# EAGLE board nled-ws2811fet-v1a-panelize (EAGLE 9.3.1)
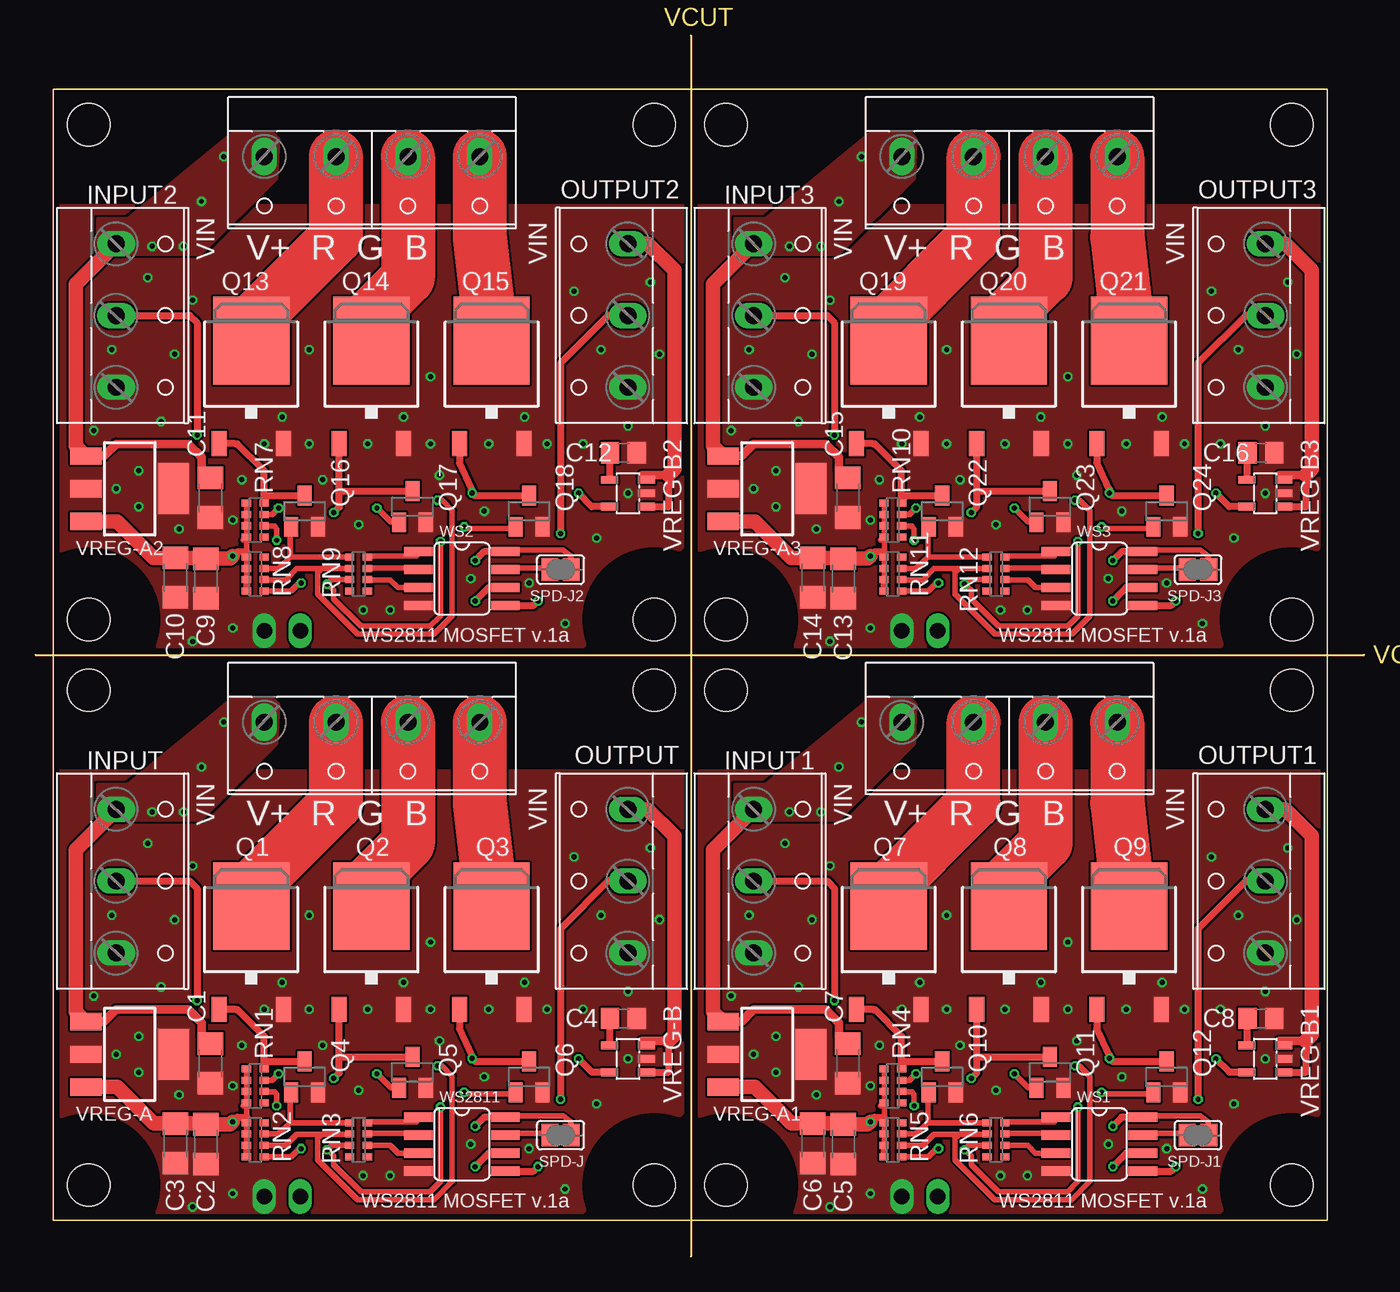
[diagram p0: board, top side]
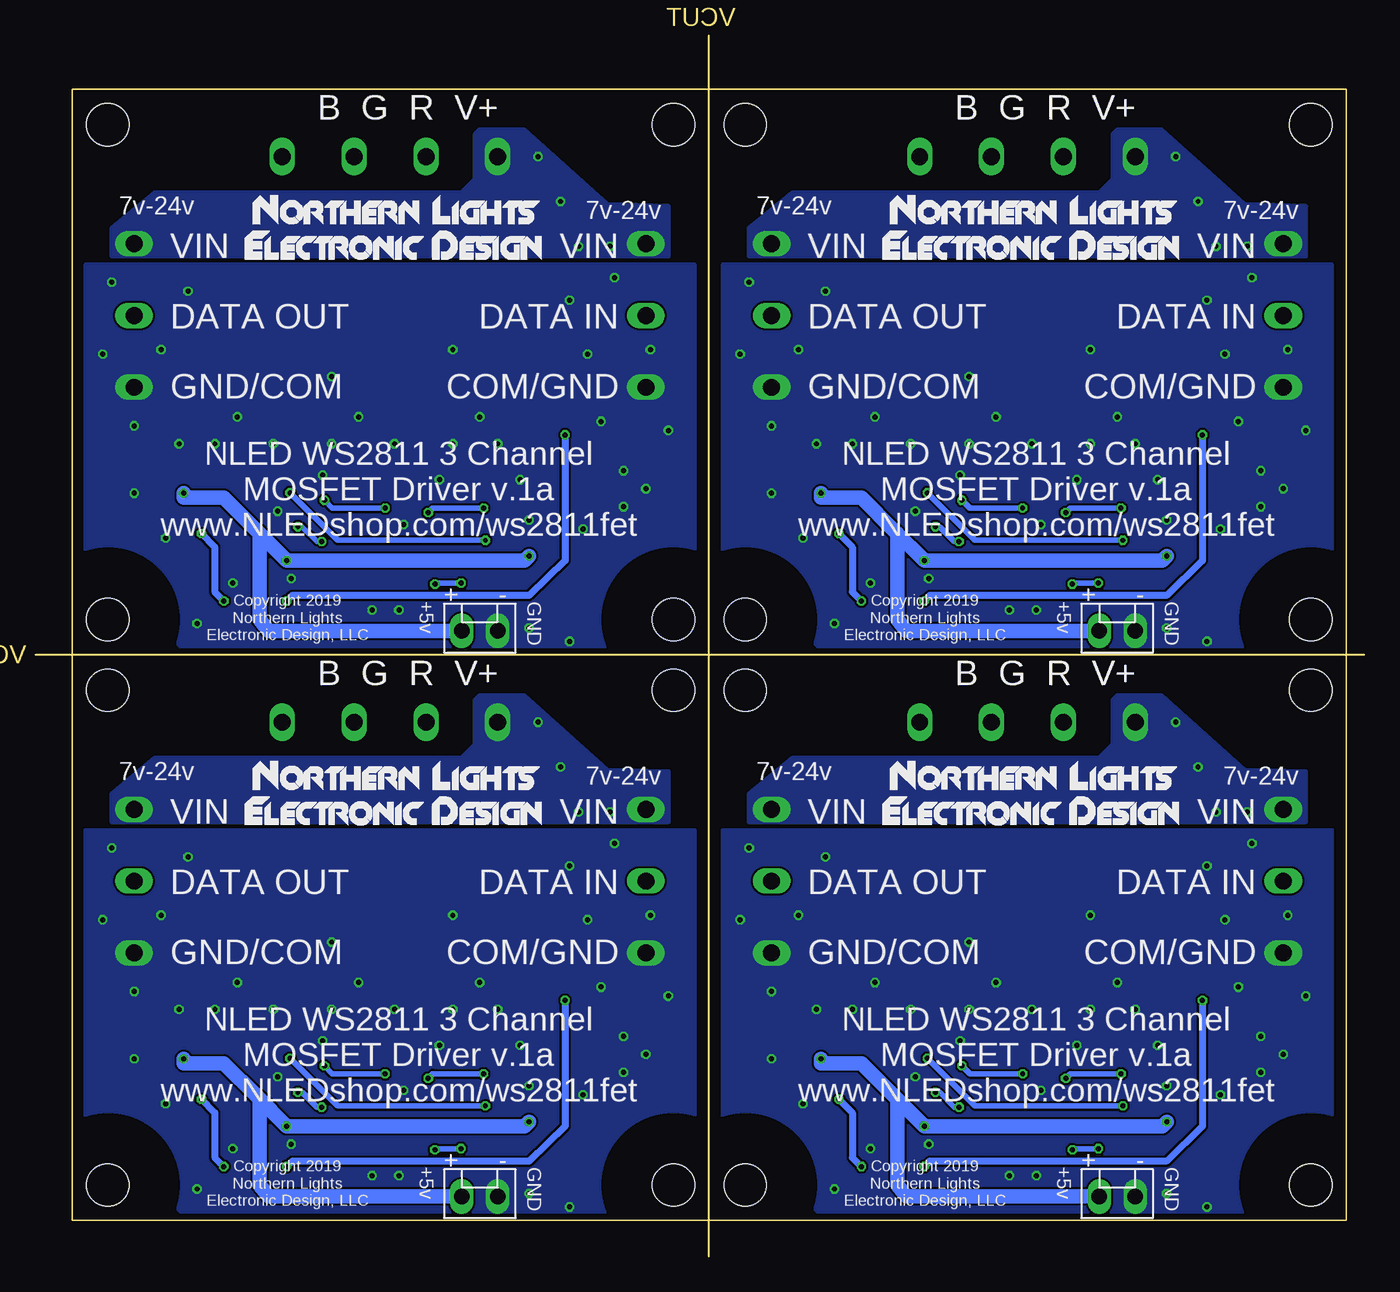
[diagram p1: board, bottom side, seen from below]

Size 93.98 x 86.36 mm. Coordinates in mm from the lower left corner, seen from the top.
Outline: 46.27,2.54 1.27,2.54 1.27,82.55
Outline: 46.36,2.54 91.35,2.54 91.35,82.55 1.27,82.55
Outline: 46.36,86.36 46.36,0
Outline: 0,42.54 93.98,42.54
Copper layers (1*2*15*16): Top 0.035mm / dielectric 0.2mm / Route2 0.0175mm / dielectric 1.1mm / Route15 0.0175mm / dielectric 0.2mm / Bottom 0.035mm
Design rules "SeeedStudio_DRU_no_angle_20130527 *": minimum track width 6mil, minimum drill 12mil, track to track 6mil, track to pad 12mil, pad to pad 6mil, via to via 6mil, smd to smd 0mil, copper to edge 16mil, drill to drill 10mil, minimum pad ring 6mil, minimum via ring 6mil, stop-mask expansion 2mil, vias tented up to drill 25mil, thermal gap 10mil
Net classes: 0 default: width 0.406 mm
Holes 3 mm at 3.77,5.04 43.77,40.04 3.77,40.04 43.77,5.04 48.86,5.04 88.85,40.04 48.86,40.04 88.85,5.04 3.77,45.05 43.77,80.05 3.77,80.05 43.77,45.05 48.86,45.05 88.85,80.05 48.86,80.05 88.85,45.05
tRestrict: area -1.2,35 to 8.8,45; area -1.2,0 to 8.8,10; area 38.8,35 to 48.8,45; area 38.8,0 to 48.8,10; area 43.9,35 to 53.9,45; area 43.9,0 to 53.9,10; area 83.9,35 to 93.9,45; area 83.9,0 to 93.9,10; area -1.2,75 to 8.8,85; area -1.2,40 to 8.8,50; area 38.8,75 to 48.8,85; area 38.8,40 to 48.8,50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
bRestrict: area -1.2,0 to 8.8,10; area -1.2,35 to 8.8,45; area 38.8,35 to 48.8,45; area 38.8,0 to 48.8,10; area 43.9,0 to 53.9,10; area 43.9,35 to 53.9,45; area 83.9,35 to 93.9,45; area 83.9,0 to 93.9,10; area -1.2,40 to 8.8,50; area -1.2,75 to 8.8,85; area 38.8,75 to 48.8,85; area 38.8,40 to 48.8,50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

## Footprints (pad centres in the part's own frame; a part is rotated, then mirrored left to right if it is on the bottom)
MOLEXKK2PWR = drill 1.1 long: 1 -1.27,0; 2 1.27,0
C1206 = smd 1.6 x 1.8: 1 -1.4,0; 2 1.4,0
C0805 = smd 1.3 x 1.5: 1 -0.95,0; 2 0.95,0
W237-133 = drill 1.194 long: 1 -5.08,-0.635; 2 0,-0.635; 3 5.08,-0.635
W237-4P = drill 1.194 long: 1 -7.62,-0.635; 2 -2.54,-0.635; 3 2.54,-0.635; 4 7.62,-0.635
DPAK-2PIN = smd 1.067 x 1.778: 1 -2.28,-6.07; 3 2.28,-6.07 | smd 5.4 x 6.2: 2 0,1.23
SOT23 = smd 1 x 1.4: 1 -0.95,-1.1; 2 0.95,-1.1; 3 0,1.1
0603-ARV = smd 0.5 x 0.65: 1 -1.2,-0.625; 2 -0.4,-0.625; 3 0.4,-0.625; 4 1.2,-0.625; 5 1.2,0.625; 6 0.4,0.625; 7 -0.4,0.625; 8 -1.2,0.625
SJ = smd 1.168 x 1.6: 1 -0.762,0; 2 0.762,0
SOT223 = smd 1.219 x 2.235: 1 -2.311,-3.099; 2 0,-3.099; 3 2.311,-3.099 | smd 3.6 x 2.2: 4 0,3.099
SOT25 = smd 0.55 x 1.2: 1 -0.95,-1.3; 2 0,-1.3; 3 0.95,-1.3; 4 0.95,1.3; 5 -0.95,1.3
SOIC-8 = smd 0.66 x 2.032: 1 -1.905,-3.073; 2 -0.635,-3.073; 3 0.635,-3.073; 4 1.905,-3.073; 5 1.905,3.073; 6 0.635,3.073; 7 -0.635,3.073; 8 -1.905,3.073

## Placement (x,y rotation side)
5VOUT  MOLEX-KK-2P5V  [MOLEXKK2PWR]  17.46,4.24 0 bottom
5VOUT1  MOLEX-KK-2P5V  [MOLEXKK2PWR]  62.55,4.24 0 bottom
5VOUT2  MOLEX-KK-2P5V  [MOLEXKK2PWR]  17.46,44.24 0 bottom
5VOUT3  MOLEX-KK-2P5V  [MOLEXKK2PWR]  62.55,44.24 0 bottom
C1  0.1uF, >24v  [C1206]  12.38,13.65 270 top
C2  0.1uF, >6.3vdc  [C1206]  12.06,7.94 270 top
C3  10uF, >6.3vdc  [C1206]  9.91,8 270 top
C4  100pF  [C0805]  41.59,16.83 0 top
C5  0.1uF, >6.3vdc  [C1206]  57.15,7.94 270 top
C6  10uF, >6.3vdc  [C1206]  54.99,8 270 top
C7  0.1uF, >24v  [C1206]  57.47,13.65 270 top
C8  100pF  [C0805]  86.68,16.83 0 top
C9  0.1uF, >6.3vdc  [C1206]  12.06,47.94 270 top
C10  10uF, >6.3vdc  [C1206]  9.91,48.01 270 top
C11  0.1uF, >24v  [C1206]  12.38,53.66 270 top
C12  100pF  [C0805]  41.59,56.83 0 top
C13  0.1uF, >6.3vdc  [C1206]  57.15,47.94 270 top
C14  10uF, >6.3vdc  [C1206]  54.99,48.01 270 top
C15  0.1uF, >24v  [C1206]  57.47,53.66 270 top
C16  100pF  [C0805]  86.68,56.83 0 top
INPUT  [W237-133]  6.35,26.54 270 top
INPUT1  [W237-133]  51.44,26.54 270 top
INPUT2  [W237-133]  6.35,66.55 270 top
INPUT3  [W237-133]  51.44,66.55 270 top
LEDOUT  [W237-4P]  23.81,37.15 180 top
LEDOUT1  [W237-4P]  68.9,37.15 180 top
LEDOUT2  [W237-4P]  23.81,77.15 180 top
LEDOUT3  [W237-4P]  68.9,77.15 180 top
OUTPUT  [W237-133]  41.28,26.54 90 top
OUTPUT1  [W237-133]  86.36,26.54 90 top
OUTPUT2  [W237-133]  41.28,66.55 90 top
OUTPUT3  [W237-133]  86.36,66.55 90 top
Q1  NCHAN-DPAK-2  [DPAK-2PIN]  15.27,23.54 0 top
Q2  NCHAN-DPAK-2  [DPAK-2PIN]  23.77,23.54 0 top
Q3  NCHAN-DPAK-2  [DPAK-2PIN]  32.27,23.54 0 top
Q4  BSS123  [SOT23]  19.05,12.7 0 top
Q5  BSS123  [SOT23]  26.67,13.02 0 top
Q6  BSS123  [SOT23]  34.93,12.7 0 top
Q7  NCHAN-DPAK-2  [DPAK-2PIN]  60.36,23.54 0 top
Q8  NCHAN-DPAK-2  [DPAK-2PIN]  68.85,23.54 0 top
Q9  NCHAN-DPAK-2  [DPAK-2PIN]  77.35,23.54 0 top
Q10  BSS123  [SOT23]  64.14,12.7 0 top
Q11  BSS123  [SOT23]  71.75,13.02 0 top
Q12  BSS123  [SOT23]  80.01,12.7 0 top
Q13  NCHAN-DPAK-2  [DPAK-2PIN]  15.27,63.55 0 top
Q14  NCHAN-DPAK-2  [DPAK-2PIN]  23.77,63.55 0 top
Q15  NCHAN-DPAK-2  [DPAK-2PIN]  32.27,63.55 0 top
Q16  BSS123  [SOT23]  19.05,52.7 0 top
Q17  BSS123  [SOT23]  26.67,53.02 0 top
Q18  BSS123  [SOT23]  34.93,52.7 0 top
Q19  NCHAN-DPAK-2  [DPAK-2PIN]  60.36,63.55 0 top
Q20  NCHAN-DPAK-2  [DPAK-2PIN]  68.85,63.55 0 top
Q21  NCHAN-DPAK-2  [DPAK-2PIN]  77.35,63.55 0 top
Q22  BSS123  [SOT23]  64.14,52.7 0 top
Q23  BSS123  [SOT23]  71.75,53.02 0 top
Q24  BSS123  [SOT23]  80.01,52.7 0 top
RN1  10k  [0603-ARV]  15.56,12.07 90 top
RN2  10k  [0603-ARV]  15.56,8.25 90 top
RN3  100  [0603-ARV]  22.86,8.25 270 top
RN4  10k  [0603-ARV]  60.64,12.07 90 top
RN5  10k  [0603-ARV]  60.64,8.25 90 top
RN6  100  [0603-ARV]  67.94,8.25 270 top
RN7  10k  [0603-ARV]  15.56,52.07 90 top
RN8  10k  [0603-ARV]  15.56,48.26 90 top
RN9  100  [0603-ARV]  22.86,48.26 270 top
RN10  10k  [0603-ARV]  60.64,52.07 90 top
RN11  10k  [0603-ARV]  60.64,48.26 90 top
RN12  100  [0603-ARV]  67.94,48.26 270 top
SPD-J  [SJ]  37.15,8.57 0 top
SPD-J1  [SJ]  82.23,8.57 0 top
SPD-J2  [SJ]  37.15,48.58 0 top
SPD-J3  [SJ]  82.23,48.58 0 top
VREG-A  UA78M05DCY  [SOT223]  6.67,14.29 270 top
VREG-A1  UA78M05DCY  [SOT223]  51.75,14.29 270 top
VREG-A2  UA78M05DCY  [SOT223]  6.67,54.29 270 top
VREG-A3  UA78M05DCY  [SOT223]  51.75,54.29 270 top
VREG-B  AP2210K  [SOT25]  41.91,13.97 90 top
VREG-B1  AP2210K  [SOT25]  86.99,13.97 90 top
VREG-B2  AP2210K  [SOT25]  41.91,53.98 90 top
VREG-B3  AP2210K  [SOT25]  86.99,53.98 90 top
WS1  WS2811  [SOIC-8]  75.25,7.94 270 top
WS2  WS2811  [SOIC-8]  30.16,47.94 270 top
WS3  WS2811  [SOIC-8]  75.25,47.94 270 top
WS2811  WS2811  [SOIC-8]  30.16,7.94 270 top

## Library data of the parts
5VOUT 5VOUT1-5VOUT3 = NLED-connectors
C1-C3 C5-C7 C9-C11 C13-C15 = rcl
C4 C8 C12 C16 = rcl; SPICEPREFIX: C
INPUT INPUT1-INPUT3 LEDOUT LEDOUT1-LEDOUT3 OUTPUT OUTPUT1-OUTPUT3 = con-wago-508; OC_FARNELL: unknown; OC_NEWARK: unknown
Q1-Q3 Q7-Q9 Q13-Q15 Q19-Q21 VREG-A VREG-A1-VREG-A3 VREG-B VREG-B1-VREG-B3 WS1-WS3 WS2811 = NLED-integratedcircuit
Q4-Q6 Q10-Q12 Q16-Q18 Q22-Q24 = transistor-small-signal
RN1-RN12 = resistor-dil; OC_FARNELL: unknown; OC_NEWARK: unknown
SPD-J SPD-J1-SPD-J3 = NLED-misc

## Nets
BINV: Q3.1 Q6.3 RN1.2
BINV1: Q9.1 Q12.3 RN4.2
BINV2: Q15.1 Q18.3 RN7.2
BINV3: Q21.1 Q24.3 RN10.2
BYPASS: C4.1 VREG-B.4
BYPASS1: C8.1 VREG-B1.4
BYPASS2: C12.1 VREG-B2.4
BYPASS3: C16.1 VREG-B3.4
DIN: INPUT.2 WS2811.6
DIN1: INPUT1.2 WS1.6
DIN2: INPUT2.2 WS2.6
DIN3: INPUT3.2 WS3.6
DOUT: OUTPUT.2 WS2811.5
DOUT1: OUTPUT1.2 WS1.5
DOUT2: OUTPUT2.2 WS2.5
DOUT3: OUTPUT3.2 WS3.5
GINV: Q2.1 Q5.3 RN1.3
GINV1: Q8.1 Q11.3 RN4.3
GINV2: Q14.1 Q17.3 RN7.3
GINV3: Q20.1 Q23.3 RN10.3
GND: 5VOUT.2 C1.2 C2.2 C3.2 C4.2 INPUT.3 OUTPUT.1 Q1.3 Q2.3 Q3.3 Q4.2 Q5.2 Q6.2 VREG-A.2 VREG-A.4 VREG-B.2 WS2811.4
GND1: 5VOUT1.2 C5.2 C6.2 C7.2 C8.2 INPUT1.3 OUTPUT1.1 Q7.3 Q8.3 Q9.3 Q10.2 Q11.2 Q12.2 VREG-A1.2 VREG-A1.4 VREG-B1.2 WS1.4
GND2: 5VOUT2.2 C9.2 C10.2 C11.2 C12.2 INPUT2.3 OUTPUT2.1 Q13.3 Q14.3 Q15.3 Q16.2 Q17.2 Q18.2 VREG-A2.2 VREG-A2.4 VREG-B2.2 WS2.4
GND3: 5VOUT3.2 C13.2 C14.2 C15.2 C16.2 INPUT3.3 OUTPUT3.1 Q19.3 Q20.3 Q21.3 Q22.2 Q23.2 Q24.2 VREG-A3.2 VREG-A3.4 VREG-B3.2 WS3.4
N$1: SPD-J1.1 WS1.7
N$2: RN6.8 WS1.1
N$3: RN3.8 WS2811.1
N$4: RN6.7 WS1.2
N$5: RN3.7 WS2811.2
N$6: RN6.6 WS1.3
N$7: RN3.6 WS2811.3
N$8: SPD-J2.1 WS2.7
N$9: RN9.8 WS2.1
N$10: RN9.7 WS2.2
N$11: RN9.6 WS2.3
N$12: SPD-J3.1 WS3.7
N$13: SPD-J.1 WS2811.7
N$14: RN12.8 WS3.1
N$15: RN12.7 WS3.2
N$16: RN12.6 WS3.3
OUTB-1: Q6.1 RN2.1 RN3.3
OUTB-2: Q12.1 RN5.1 RN6.3
OUTB-3: Q18.1 RN8.1 RN9.3
OUTB-4: Q24.1 RN11.1 RN12.3
OUTBLUE: LEDOUT.3 Q1.2
OUTBLUE1: LEDOUT1.3 Q7.2
OUTBLUE2: LEDOUT2.3 Q13.2
OUTBLUE3: LEDOUT3.3 Q19.2
OUTG-1: Q5.1 RN2.2 RN3.2
OUTG-2: Q11.1 RN5.2 RN6.2
OUTG-3: Q17.1 RN8.2 RN9.2
OUTG-4: Q23.1 RN11.2 RN12.2
OUTGREEN: LEDOUT.2 Q2.2
OUTGREEN1: LEDOUT1.2 Q8.2
OUTGREEN2: LEDOUT2.2 Q14.2
OUTGREEN3: LEDOUT3.2 Q20.2
OUTR-1: Q4.1 RN2.3 RN3.1
OUTR-2: Q10.1 RN5.3 RN6.1
OUTR-3: Q16.1 RN8.3 RN9.1
OUTR-4: Q22.1 RN11.3 RN12.1
OUTRED: LEDOUT.1 Q3.2
OUTRED1: LEDOUT1.1 Q9.2
OUTRED2: LEDOUT2.1 Q15.2
OUTRED3: LEDOUT3.1 Q21.2
RINV: Q1.1 Q4.3 RN1.4
RINV1: Q7.1 Q10.3 RN4.4
RINV2: Q13.1 Q16.3 RN7.4
RINV3: Q19.1 Q22.3 RN10.4
VCC: 5VOUT.1 C2.1 C3.1 RN1.5 RN1.6 RN1.7 RN1.8 RN2.5 RN2.6 RN2.7 RN2.8 SPD-J.2 VREG-A.3 VREG-B.5 WS2811.8
VCC1: 5VOUT1.1 C5.1 C6.1 RN4.5 RN4.6 RN4.7 RN4.8 RN5.5 RN5.6 RN5.7 RN5.8 SPD-J1.2 VREG-A1.3 VREG-B1.5 WS1.8
VCC2: 5VOUT2.1 C9.1 C10.1 RN7.5 RN7.6 RN7.7 RN7.8 RN8.5 RN8.6 RN8.7 RN8.8 SPD-J2.2 VREG-A2.3 VREG-B2.5 WS2.8
VCC3: 5VOUT3.1 C13.1 C14.1 RN10.5 RN10.6 RN10.7 RN10.8 RN11.5 RN11.6 RN11.7 RN11.8 SPD-J3.2 VREG-A3.3 VREG-B3.5 WS3.8
VIN: C1.1 INPUT.1 LEDOUT.4 OUTPUT.3 VREG-A.1 VREG-B.1 VREG-B.3
VIN1: C7.1 INPUT1.1 LEDOUT1.4 OUTPUT1.3 VREG-A1.1 VREG-B1.1 VREG-B1.3
VIN2: C11.1 INPUT2.1 LEDOUT2.4 OUTPUT2.3 VREG-A2.1 VREG-B2.1 VREG-B2.3
VIN3: C15.1 INPUT3.1 LEDOUT3.4 OUTPUT3.3 VREG-A3.1 VREG-B3.1 VREG-B3.3

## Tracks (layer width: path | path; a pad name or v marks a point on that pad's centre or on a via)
BINV  (via drill 0.35)
  Top 0.406: RN1.2 16.32,11.64 16.92,11.64 17.07,11.45 v17.07,10.64
  Top 0.508: Q3.1 29.99,16.13 30.89,14.23 v30.89,14 31.08,13.8 Q6.3
  Bottom 0.406: v17.07,10.64 27.53,10.64 v30.89,14
BINV1  (via drill 0.35)
  Top 0.406: RN4.2 61.4,11.64 62,11.64 62.16,11.45 v62.16,10.64
  Top 0.508: Q9.1 75.08,16.13 75.97,14.23 v75.97,14 76.17,13.8 Q12.3
  Bottom 0.406: v62.16,10.64 72.62,10.64 v75.97,14
BINV2  (via drill 0.35)
  Top 0.406: RN7.2 16.32,51.64 16.92,51.64 17.07,51.45 v17.07,50.65
  Top 0.508: Q15.1 29.99,56.13 30.89,54.23 v30.89,54 31.08,53.8 Q18.3
  Bottom 0.406: v17.07,50.65 27.53,50.65 v30.89,54
BINV3  (via drill 0.35)
  Top 0.406: RN10.2 61.4,51.64 62,51.64 62.16,51.45 v62.16,50.65
  Top 0.508: Q21.1 75.08,56.13 75.97,54.23 v75.97,54 76.17,53.8 Q24.3
  Bottom 0.406: v62.16,50.65 72.62,50.65 v75.97,54
BYPASS
  Top 0.508: VREG-B.4 40.64,14.95 C4.1
BYPASS1
  Top 0.508: VREG-B1.4 85.73,14.95 C8.1
BYPASS2
  Top 0.508: VREG-B2.4 40.64,54.96 C12.1
BYPASS3
  Top 0.508: VREG-B3.4 85.73,54.96 C16.1
DIN  (via drill 0.35)
  Top 0.508: WS2811.6 32.07,7.3 v31.11,6.35 | v11.43,18.1 11.43,26.04 10.92,26.54 INPUT.2
  Bottom 0.508: v11.43,18.1 11.43,9.21 13.97,6.74 26.35,6.74 30.72,6.74 v31.11,6.35
DIN1  (via drill 0.35)
  Top 0.508: WS1.6 77.15,7.3 v76.2,6.35 | v56.52,18.1 56.52,26.04 56.01,26.54 INPUT1.2
  Bottom 0.508: v56.52,18.1 56.52,9.21 59.05,6.74 71.44,6.74 75.81,6.74 v76.2,6.35
DIN2  (via drill 0.35)
  Top 0.508: WS2.6 32.07,47.31 v31.11,46.35 | v11.43,58.1 11.43,66.04 10.92,66.55 INPUT2.2
  Bottom 0.508: v11.43,58.1 11.43,49.21 13.97,46.74 26.35,46.74 30.72,46.74 v31.11,46.35
DIN3  (via drill 0.35)
  Top 0.508: WS3.6 77.15,47.31 v76.2,46.35 | v56.52,58.1 56.52,66.04 56.01,66.55 INPUT3.2
  Bottom 0.508: v56.52,58.1 56.52,49.21 59.05,46.74 71.44,46.74 75.81,46.74 v76.2,46.35
DOUT  (via drill 0.35)
  Top 0.508: WS2811.5 35.24,6.03 v35.56,6.35 | OUTPUT.2 40.51,26.54 37.15,23.18 v37.15,11.11
  Bottom 0.508: v35.56,6.35 36.2,6.99 36.2,10.16 v37.15,11.11
DOUT1  (via drill 0.35)
  Top 0.508: WS1.5 80.33,6.03 v80.64,6.35 | OUTPUT1.2 85.59,26.54 82.23,23.18 v82.23,11.11
  Bottom 0.508: v80.64,6.35 81.28,6.99 81.28,10.16 v82.23,11.11
DOUT2  (via drill 0.35)
  Top 0.508: WS2.5 35.24,46.04 v35.56,46.35 | OUTPUT2.2 40.51,66.55 37.15,63.18 v37.15,51.12
  Bottom 0.508: v35.56,46.35 36.2,46.99 36.2,50.16 v37.15,51.12
DOUT3  (via drill 0.35)
  Top 0.508: WS3.5 80.33,46.04 v80.64,46.35 | OUTPUT3.2 85.59,66.55 82.23,63.18 v82.23,51.12
  Bottom 0.508: v80.64,46.35 81.28,46.99 81.28,50.16 v82.23,51.12
GINV  (via drill 0.35)
  Top 0.406: v17.2,12.92 16.75,12.46 RN1.3
  Top 0.508: v21.11,12.6 21.49,12.98 21.49,13.97 | 21.49,13.97 Q2.1 | 21.49,13.97 21.64,14.12 Q5.3
  Bottom 0.406: v21.11,12.6 20.79,12.92 v17.2,12.92
GINV1  (via drill 0.35)
  Top 0.406: v62.28,12.92 61.83,12.46 RN4.3
  Top 0.508: v66.19,12.6 66.58,12.98 66.58,13.97 | 66.58,13.97 Q8.1 | 66.58,13.97 66.72,14.12 Q11.3
  Bottom 0.406: v66.19,12.6 65.88,12.92 v62.28,12.92
GINV2  (via drill 0.35)
  Top 0.406: v17.2,52.92 16.75,52.47 RN7.3
  Top 0.508: v21.11,52.6 21.49,52.99 21.49,53.98 | 21.49,53.98 Q14.1 | 21.49,53.98 21.64,54.12 Q17.3
  Bottom 0.406: v21.11,52.6 20.79,52.92 v17.2,52.92
GINV3  (via drill 0.35)
  Top 0.406: v62.28,52.92 61.83,52.47 RN10.3
  Top 0.508: v66.19,52.6 66.58,52.99 66.58,53.98 | 66.58,53.98 Q20.1 | 66.58,53.98 66.72,54.12 Q23.3
  Bottom 0.406: v66.19,52.6 65.88,52.92 v62.28,52.92
GND  (via drill 0.35)
  other vias: 19.37,24.13 5.4,24.13 20.32,14.92 11.11,3.49 4.13,18.41 5.71,14.29 38.1,28.26 11.11,27.62 39.69,10.8 38.74,17.46 13.97,4.45 23.18,5.71 25.08,5.71 22.86,11.75 28.57,15.24 31.75,12.7 40.01,24.13 41.91,13.97 27.94,22.22 41.91,18.73 14.61,14.92 10.16,11.43 7.3,13.02 8.89,19.05 9.84,23.81 23.5,17.46 27.94,17.46 16.19,17.46 32.07,17.46 36.2,17.46 34.61,19.37 26.04,19.37 17.46,19.37 19.37,17.46 34.93,7.62 30.8,7.94 13.97,12.07 7.3,15.56 7.94,29.21 43.5,28.89 44.13,23.81 37.47,4.76
  pour Top (rank 2, no thermals): 1.27,34.29 46.36,34.29 46.36,10.8 38.1,2.54 8.89,2.54 1.27,10.16
  pour Bottom (rank 2, no thermals): 2.22,30.16 45.4,30.16 45.4,9.84 38.1,2.54 8.89,2.54 2.22,9.21
GND1  (via drill 0.35)
  other vias: 64.45,24.13 50.48,24.13 65.41,14.92 56.2,3.49 49.21,18.41 50.8,14.29 83.19,28.26 56.2,27.62 84.77,10.8 83.82,17.46 59.05,4.45 68.26,5.71 70.17,5.71 67.94,11.75 73.66,15.24 76.83,12.7 85.09,24.13 86.99,13.97 73.02,22.22 86.99,18.73 59.69,14.92 55.25,11.43 52.39,13.02 53.98,19.05 54.93,23.81 68.58,17.46 73.02,17.46 61.28,17.46 77.15,17.46 81.28,17.46 79.69,19.37 71.12,19.37 62.55,19.37 64.45,17.46 80.01,7.62 75.88,7.94 59.05,12.07 52.39,15.56 53.02,29.21 88.58,28.89 89.22,23.81 82.55,4.76
  pour Top (rank 2, no thermals): 46.36,34.29 91.44,34.29 91.44,10.8 83.19,2.54 53.98,2.54 46.36,10.16
  pour Bottom (rank 2, no thermals): 47.31,30.16 90.49,30.16 90.49,9.84 83.19,2.54 53.98,2.54 47.31,9.21
GND2  (via drill 0.35)
  other vias: 19.37,64.14 5.4,64.14 20.32,54.93 11.11,43.5 4.13,58.42 5.71,54.29 38.1,68.26 11.11,67.63 39.69,50.8 38.74,57.47 13.97,44.45 23.18,45.72 25.08,45.72 22.86,51.75 28.57,55.24 31.75,52.7 40.01,64.14 41.91,53.98 27.94,62.23 41.91,58.74 14.61,54.93 10.16,51.44 7.3,53.02 8.89,59.05 9.84,63.82 23.5,57.47 27.94,57.47 16.19,57.47 32.07,57.47 36.2,57.47 34.61,59.37 26.04,59.37 17.46,59.37 19.37,57.47 34.93,47.62 30.8,47.94 13.97,52.07 7.3,55.56 7.94,69.22 43.5,68.9 44.13,63.82 37.47,44.77
  pour Top (rank 2, no thermals): 1.27,74.3 46.36,74.3 46.36,50.8 38.1,42.55 8.89,42.55 1.27,50.16
  pour Bottom (rank 2, no thermals): 2.22,70.17 45.4,70.17 45.4,49.85 38.1,42.55 8.89,42.55 2.22,49.21
GND3  (via drill 0.35)
  other vias: 64.45,64.14 50.48,64.14 65.41,54.93 56.2,43.5 49.21,58.42 50.8,54.29 83.19,68.26 56.2,67.63 84.77,50.8 83.82,57.47 59.05,44.45 68.26,45.72 70.17,45.72 67.94,51.75 73.66,55.24 76.83,52.7 85.09,64.14 86.99,53.98 73.02,62.23 86.99,58.74 59.69,54.93 55.25,51.44 52.39,53.02 53.98,59.05 54.93,63.82 68.58,57.47 73.02,57.47 61.28,57.47 77.15,57.47 81.28,57.47 79.69,59.37 71.12,59.37 62.55,59.37 64.45,57.47 80.01,47.62 75.88,47.94 59.05,52.07 52.39,55.56 53.02,69.22 88.58,68.9 89.22,63.82 82.55,44.77
  pour Top (rank 2, no thermals): 46.36,74.3 91.44,74.3 91.44,50.8 83.19,42.55 53.98,42.55 46.36,50.16
  pour Bottom (rank 2, no thermals): 47.31,70.17 90.49,70.17 90.49,49.85 83.19,42.55 53.98,42.55 47.31,49.21
N$1
  Top 0.406: SPD-J1.1 81.36,8.69 78.49,8.69 WS1.7
N$2
  Top 0.406: RN6.8 68.71,9.53 72.06,9.53 WS1.1
N$3
  Top 0.406: RN3.8 23.62,9.53 26.97,9.53 WS2811.1
N$4
  Top 0.406: RN6.7 68.71,8.69 72.06,8.69 WS1.2
N$5
  Top 0.406: RN3.7 23.62,8.69 26.97,8.69 WS2811.2
N$6
  Top 0.406: WS1.3 70.74,7.3 70.19,7.85 68.71,7.85 RN6.6
N$7
  Top 0.406: WS2811.3 25.65,7.3 25.11,7.85 23.62,7.85 RN3.6
N$8
  Top 0.406: SPD-J2.1 36.28,48.69 33.4,48.69 WS2.7
N$9
  Top 0.406: RN9.8 23.62,49.53 26.97,49.53 WS2.1
N$10
  Top 0.406: RN9.7 23.62,48.69 26.97,48.69 WS2.2
N$11
  Top 0.406: WS2.3 25.65,47.31 25.11,47.85 23.62,47.85 RN9.6
N$12
  Top 0.406: SPD-J3.1 81.36,48.69 78.49,48.69 WS3.7
N$13
  Top 0.406: SPD-J.1 36.28,8.69 33.4,8.69 WS2811.7
N$14
  Top 0.406: RN12.8 68.71,49.53 72.06,49.53 WS3.1
N$15
  Top 0.406: RN12.7 68.71,48.69 72.06,48.69 WS3.2
N$16
  Top 0.406: WS3.3 70.74,47.31 70.19,47.85 68.71,47.85 RN12.6
OUTB-1  (via drill 0.35)
  Top 0.406: 33.96,11.48 Q6.1 33.96,11.48 | v18.8,7.62 18.79,7.76 18.09,7.05 RN2.1 | RN3.3 20.95,7.86 v20.64,7.54 21.11,7.12 21.11,6.49 23.02,4.57 27.93,4.57 28.65,5.3 v28.65,10.55 | 33.96,11.48 30.33,11.48 v30.33,11.59
  Bottom 0.406: v20.64,7.54 20.64,7.44 20.62,7.62 v18.8,7.62 | v30.33,11.59 30.01,11.59 28.97,10.55 v28.65,10.55
OUTB-2  (via drill 0.35)
  Top 0.406: 79.05,11.48 Q12.1 79.05,11.48 | v63.88,7.62 63.88,7.76 63.17,7.05 RN5.1 | RN6.3 66.04,7.86 v65.72,7.54 66.19,7.12 66.19,6.49 68.11,4.57 73.01,4.57 73.74,5.3 v73.74,10.55 | 79.05,11.48 75.41,11.48 v75.41,11.59
  Bottom 0.406: v65.72,7.54 65.72,7.44 65.71,7.62 v63.88,7.62 | v75.41,11.59 75.09,11.59 74.05,10.55 v73.74,10.55
OUTB-3  (via drill 0.35)
  Top 0.406: 33.96,51.49 Q18.1 33.96,51.49 | v18.8,47.62 18.79,47.77 18.09,47.06 RN8.1 | RN9.3 20.95,47.86 v20.64,47.55 21.11,47.12 21.11,46.49 23.02,44.58 27.93,44.58 28.65,45.3 v28.65,50.56 | 33.96,51.49 30.33,51.49 v30.33,51.6
  Bottom 0.406: v20.64,47.55 20.64,47.45 20.62,47.62 v18.8,47.62 | v30.33,51.6 30.01,51.6 28.97,50.56 v28.65,50.56
OUTB-4  (via drill 0.35)
  Top 0.406: 79.05,51.49 Q24.1 79.05,51.49 | v63.88,47.62 63.88,47.77 63.17,47.06 RN11.1 | RN12.3 66.04,47.86 v65.72,47.55 66.19,47.12 66.19,46.49 68.11,44.58 73.01,44.58 73.74,45.3 v73.74,50.56 | 79.05,51.49 75.41,51.49 v75.41,51.6
  Bottom 0.406: v65.72,47.55 65.72,47.45 65.71,47.62 v63.88,47.62 | v75.41,51.6 75.09,51.6 74.05,50.56 v73.74,50.56
OUTBLUE
  Top 2.54: Q1.2 15.56,24.92 14.61,25.4
  Top 3.81: 14.61,25.4 21.27,32.07 LEDOUT.3
OUTBLUE1
  Top 2.54: Q7.2 60.64,24.92 59.69,25.4
  Top 3.81: 59.69,25.4 66.36,32.07 LEDOUT1.3
OUTBLUE2
  Top 2.54: Q13.2 15.56,64.93 14.61,65.41
  Top 3.81: 14.61,65.41 21.27,72.07 LEDOUT2.3
OUTBLUE3
  Top 2.54: Q19.2 60.64,64.93 59.69,65.41
  Top 3.81: 59.69,65.41 66.36,72.07 LEDOUT3.3
OUTG-1  (via drill 0.35)
  Top 0.406: RN2.2 16.25,7.84 17.69,7.84 18.48,8.64 20.32,8.64 | v24.16,12.92 25.15,11.92 Q5.1 | v28.45,13.48 28.77,13.48 29.49,12.75 29.49,5.3 28.21,4.01 22.78,4.01 19.95,6.84 19.95,8.35 20.32,8.64 | 20.32,8.64 21.59,8.64 | 21.59,8.64 21.99,8.64 | 21.59,8.64 RN3.2
  Bottom 0.406: v24.16,12.92 27.89,12.92 v28.45,13.48
OUTG-2  (via drill 0.35)
  Top 0.406: RN5.2 61.34,7.84 62.78,7.84 63.57,8.64 65.41,8.64 | v69.24,12.92 70.24,11.92 Q11.1 | v73.53,13.48 73.85,13.48 74.57,12.75 74.57,5.3 73.29,4.01 67.87,4.01 65.04,6.84 65.04,8.35 65.41,8.64 | 65.41,8.64 66.67,8.64 | 66.67,8.64 67.08,8.64 | 66.67,8.64 RN6.2
  Bottom 0.406: v69.24,12.92 72.97,12.92 v73.53,13.48
OUTG-3  (via drill 0.35)
  Top 0.406: RN8.2 16.25,47.84 17.69,47.84 18.48,48.64 20.32,48.64 | v24.16,52.92 25.15,51.92 Q17.1 | v28.45,53.48 28.77,53.48 29.49,52.76 29.49,45.3 28.21,44.02 22.78,44.02 19.95,46.85 19.95,48.35 20.32,48.64 | 20.32,48.64 21.59,48.64 | 21.59,48.64 21.99,48.64 | 21.59,48.64 RN9.2
  Bottom 0.406: v24.16,52.92 27.89,52.92 v28.45,53.48
OUTG-4  (via drill 0.35)
  Top 0.406: RN11.2 61.34,47.84 62.78,47.84 63.57,48.64 65.41,48.64 | v69.24,52.92 70.24,51.92 Q23.1 | v73.53,53.48 73.85,53.48 74.57,52.76 74.57,45.3 73.29,44.02 67.87,44.02 65.04,46.85 65.04,48.35 65.41,48.64 | 65.41,48.64 66.67,48.64 | 66.67,48.64 67.08,48.64 | 66.67,48.64 RN12.2
  Bottom 0.406: v69.24,52.92 72.97,52.92 v73.53,53.48
OUTGREEN
  Top 3.81: LEDOUT.2 26.35,29.21 23.49,26.35 23.48,24.06 Q2.2
OUTGREEN1
  Top 3.81: LEDOUT1.2 71.44,29.21 68.58,26.35 68.57,24.06 Q8.2
OUTGREEN2
  Top 3.81: LEDOUT2.2 26.35,69.22 23.49,66.35 23.48,64.06 Q14.2
OUTGREEN3
  Top 3.81: LEDOUT3.2 71.44,69.22 68.58,66.35 68.57,64.06 Q20.2
OUTR-1
  Top 0.406: 18.03,9.44 17.16,8.66 RN2.3 | 18.03,9.44 18.03,11.48 Q4.1 | 18.03,9.44 21.95,9.44 RN3.1
OUTR-2
  Top 0.406: 63.12,9.44 62.25,8.66 RN5.3 | 63.12,9.44 63.12,11.48 Q10.1 | 63.12,9.44 67.03,9.44 RN6.1
OUTR-3
  Top 0.406: 18.03,49.45 17.16,48.66 RN8.3 | 18.03,49.45 18.03,51.49 Q16.1 | 18.03,49.45 21.95,49.45 RN9.1
OUTR-4
  Top 0.406: 63.12,49.45 62.25,48.66 RN11.3 | 63.12,49.45 63.12,51.49 Q22.1 | 63.12,49.45 67.03,49.45 RN12.1
OUTRED
  Top 3.81: LEDOUT.1 31.43,32.07 Q3.2
OUTRED1
  Top 3.81: LEDOUT1.1 76.52,32.07 Q9.2
OUTRED2
  Top 3.81: LEDOUT2.1 31.43,72.07 Q15.2
OUTRED3
  Top 3.81: LEDOUT3.1 76.52,72.07 Q21.2
RINV
  Top 0.508: Q1.1 14.14,17.47 14.25,17.42 14.29,17.46 16.18,15.57 RN1.4 16.18,13.58 16.4,13.8 Q4.3
RINV1
  Top 0.508: Q7.1 59.23,17.47 59.33,17.42 59.37,17.46 61.27,15.57 RN4.4 61.27,13.58 61.49,13.8 Q10.3
RINV2
  Top 0.508: Q13.1 14.14,57.48 14.25,57.43 14.29,57.47 16.18,55.57 RN7.4 16.18,53.59 16.4,53.8 Q16.3
RINV3
  Top 0.508: Q19.1 59.23,57.48 59.33,57.43 59.37,57.47 61.27,55.57 RN10.4 61.27,53.59 61.49,53.8 Q22.3
VCC  (via drill 0.35)
  Top 0.406: 14.96,7.01 14.93,7.04 RN2.8 | RN2.7 14.95,7.86 14.96,7.85 14.96,8.48 RN2.6 14.96,8.68 14.96,8.69 14.96,9.32 RN2.5 14.96,9.6 14.96,9.84 14.96,10.64 RN1.8 | RN1.8 14.96,10.92 14.96,11.48 RN1.7 14.96,11.76 14.96,12.32 RN1.6 14.96,12.6 14.96,13.16 RN1.5 | 14.68,10.64 RN1.8 | SPD-J.2 37.87,8.65 37.87,9.53 37.31,9.94 33.4,9.94 WS2811.8
  Top 0.508: v13.97,9.53 14.29,9.84 14.96,9.84 | WS2811.8 31.75,9.84 v31.11,9.21 | VREG-B.5 39.35,13.02 39.34,13.02 39.34,13.05 v38.42,13.97 | RN2.7 RN2.8
  Top 1.016: 12,9.4 C2.1 13.78,9.34 v13.97,9.53 | 12,9.4 C3.1 | VREG-A.3 5.8,11.98 8.38,9.4 12,9.4
  Bottom 1.016: v13.97,9.53 14.29,9.21 v31.11,9.21 33.18,11.27 | 33.18,11.27 35.56,13.65 38.42,13.65 v38.42,13.97 | 5VOUT.1 32.38,4.24 33.02,5.03 33.02,11.11 33.18,11.27
VCC1  (via drill 0.35)
  Top 0.406: 60.05,7.01 60.02,7.04 RN5.8 | RN5.7 60.05,7.85 60.05,8.48 RN5.6 60.04,8.68 60.05,8.69 60.05,9.32 RN5.5 60.05,9.6 60.05,9.84 60.05,10.64 RN4.8 | RN4.8 60.05,10.92 60.05,11.48 RN4.7 60.05,11.76 60.05,12.32 RN4.6 60.05,12.6 60.05,13.16 RN4.5 | 59.77,10.64 RN4.8 | SPD-J1.2 82.96,8.65 82.96,9.53 82.4,9.94 78.49,9.94 WS1.8
  Top 0.508: v59.05,9.53 59.37,9.84 60.05,9.84 | WS1.8 76.83,9.84 v76.2,9.21 | VREG-B1.5 84.43,13.02 84.43,13.05 v83.5,13.97 | RN5.7 RN5.8
  Top 1.016: 57.09,9.4 C5.1 58.87,9.34 v59.05,9.53 | 57.09,9.4 C6.1 | VREG-A1.3 50.89,11.98 53.46,9.4 57.09,9.4
  Bottom 1.016: v59.05,9.53 59.37,9.21 v76.2,9.21 78.26,11.27 | 78.26,11.27 80.64,13.65 83.5,13.65 v83.5,13.97 | 5VOUT1.1 77.47,4.24 78.1,5.03 78.1,11.11 78.26,11.27
VCC2  (via drill 0.35)
  Top 0.406: 14.96,47.02 14.93,47.04 RN8.8 | RN8.7 14.95,47.86 14.96,47.85 14.96,48.49 RN8.6 14.96,48.69 14.96,49.33 RN8.5 14.96,49.61 14.96,49.85 14.96,50.65 RN7.8 | RN7.8 14.96,50.93 14.96,51.49 RN7.7 14.96,51.77 14.96,52.32 RN7.6 14.96,52.6 14.96,53.16 RN7.5 | 14.68,50.65 RN7.8 | SPD-J2.2 37.87,48.65 37.87,49.53 37.31,49.95 33.4,49.95 WS2.8
  Top 0.508: v13.97,49.53 14.29,49.85 14.96,49.85 | WS2.8 31.75,49.85 v31.11,49.21 | VREG-B2.5 39.35,53.02 39.34,53.02 39.34,53.05 v38.42,53.98 | RN8.7 RN8.8
  Top 1.016: 12,49.41 C9.1 13.78,49.34 v13.97,49.53 | 12,49.41 C10.1 | VREG-A2.3 5.8,51.98 8.38,49.41 12,49.41
  Bottom 1.016: v13.97,49.53 14.29,49.21 v31.11,49.21 33.18,51.28 | 33.18,51.28 35.56,53.66 38.42,53.66 v38.42,53.98 | 5VOUT2.1 32.38,44.24 33.02,45.04 33.02,51.12 33.18,51.28
VCC3  (via drill 0.35)
  Top 0.406: 60.05,47.02 60.02,47.04 RN11.8 | RN11.7 60.05,47.85 60.05,48.49 RN11.6 60.04,48.69 60.05,48.69 60.05,49.33 RN11.5 60.05,49.61 60.05,49.85 60.05,50.65 RN10.8 | RN10.8 60.05,50.93 60.05,51.49 RN10.7 60.05,51.77 60.05,52.32 RN10.6 60.05,52.6 60.05,53.16 RN10.5 | 59.77,50.65 RN10.8 | SPD-J3.2 82.96,48.65 82.96,49.53 82.4,49.95 78.49,49.95 WS3.8
  Top 0.508: v59.05,49.53 59.37,49.85 60.05,49.85 | WS3.8 76.83,49.85 v76.2,49.21 | VREG-B3.5 84.43,53.02 84.43,53.05 v83.5,53.98 | RN11.7 RN11.8
  Top 1.016: 57.09,49.41 C13.1 58.87,49.34 v59.05,49.53 | 57.09,49.41 C14.1 | VREG-A3.3 50.89,51.98 53.46,49.41 57.09,49.41
  Bottom 1.016: v59.05,49.53 59.37,49.21 v76.2,49.21 78.26,51.28 | 78.26,51.28 80.64,53.66 83.5,53.66 v83.5,53.98 | 5VOUT3.1 77.47,44.24 78.1,45.04 78.1,51.12 78.26,51.28
VIN  (via drill 0.35)
  Top 0.508: VREG-B.1 44.77,13.02 44.77,15.24 | VREG-B.3 42.9,15.24
  Top 0.61: 42.9,15.24 44.77,15.24 | VREG-A.1 4.85,16.6 5.71,17.46 10.79,17.46 11.75,16.51 11.75,15.56 12.25,15.05 C1.1
  Top 1.016: OUTPUT.3 43.31,31.62 45.19,29.74 45.19,15.66 44.77,15.24 | INPUT.1 2.86,28.76 2.86,17.31 VREG-A.1
  other vias: 13.33,37.78 10.48,31.43 11.75,34.61 8.26,31.43
  pour Top (no thermals): 4.45,33.34 6.58,33.34 13.97,39.41 16.82,39.37 17.17,39.02 17.04,36.27 11.66,30.9 4.45,30.9
  pour Bottom (no thermals): 4.13,30.72 4.13,34.29 8.47,34.41 14.33,39.69 17.46,39.69 17.78,39.37 17.78,36.2 18.73,35.24 40.45,35.24 43.5,32.7 43.5,30.72
VIN1  (via drill 0.35)
  Top 0.508: VREG-B1.1 89.85,13.02 89.85,15.24 | VREG-B1.3 87.98,15.24
  Top 0.61: 87.98,15.24 89.85,15.24 | VREG-A1.1 49.94,16.6 50.8,17.46 55.88,17.46 56.83,16.51 56.83,15.56 57.34,15.05 C7.1
  Top 1.016: OUTPUT1.3 88.39,31.62 90.27,29.74 90.27,15.66 89.85,15.24 | INPUT1.1 47.94,28.76 47.94,17.31 VREG-A1.1
  other vias: 58.42,37.78 55.56,31.43 56.83,34.61 53.34,31.43
  pour Top (no thermals): 49.53,33.34 51.67,33.34 59.05,39.41 61.91,39.37 62.25,39.02 62.13,36.27 56.75,30.9 49.53,30.9
  pour Bottom (no thermals): 49.21,30.72 49.21,34.29 53.55,34.41 59.42,39.69 62.55,39.69 62.87,39.37 62.87,36.2 63.82,35.24 85.53,35.24 88.58,32.7 88.58,30.72
VIN2  (via drill 0.35)
  Top 0.508: VREG-B2.1 44.77,53.02 44.77,55.24 | VREG-B2.3 42.9,55.24
  Top 0.61: 42.9,55.24 44.77,55.24 | VREG-A2.1 4.85,56.6 5.71,57.47 10.79,57.47 11.75,56.52 11.75,55.56 12.25,55.06 C11.1
  Top 1.016: OUTPUT2.3 43.31,71.62 45.19,69.74 45.19,55.67 44.77,55.24 | INPUT2.1 2.86,68.77 2.86,57.31 VREG-A2.1
  other vias: 13.33,77.79 10.48,71.44 11.75,74.61 8.26,71.44
  pour Top (no thermals): 4.45,73.34 6.58,73.34 13.97,79.42 16.82,79.38 17.17,79.03 17.04,76.28 11.66,70.91 4.45,70.91
  pour Bottom (no thermals): 4.13,70.73 4.13,74.3 8.47,74.42 14.33,79.69 17.46,79.69 17.78,79.38 17.78,76.2 18.73,75.25 40.45,75.25 43.5,72.71 43.5,70.73
VIN3  (via drill 0.35)
  Top 0.508: VREG-B3.1 89.85,53.02 89.85,55.24 | VREG-B3.3 87.98,55.24
  Top 0.61: 87.98,55.24 89.85,55.24 | VREG-A3.1 49.94,56.6 50.8,57.47 55.88,57.47 56.83,56.52 56.83,55.56 57.34,55.06 C15.1
  Top 1.016: OUTPUT3.3 88.39,71.62 90.27,69.74 90.27,55.67 89.85,55.24 | INPUT3.1 47.94,68.77 47.94,57.31 VREG-A3.1
  other vias: 58.42,77.79 55.56,71.44 56.83,74.61 53.34,71.44
  pour Top (no thermals): 49.53,73.34 51.67,73.34 59.05,79.42 61.91,79.38 62.25,79.03 62.13,76.28 56.75,70.91 49.53,70.91
  pour Bottom (no thermals): 49.21,70.73 49.21,74.3 53.55,74.42 59.42,79.69 62.55,79.69 62.87,79.38 62.87,76.2 63.82,75.25 85.53,75.25 88.58,72.71 88.58,70.73

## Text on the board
Dimension: VCUT | VCUT
tNames: VIN | V+ R G B | VIN | VIN | V+ R G B | VIN | WS2811 MOSFET v.1a | WS2811 MOSFET v.1a | VIN | V+ R G B | VIN | VIN | V+ R G B | VIN | WS2811 MOSFET v.1a | WS2811 MOSFET v.1a
bNames: B G R V+ | B G R V+ | 7v-24v | 7v-24v | 7v-24v | 7v-24v | VIN / DATA IN / COM/GND | VIN / DATA OUT / GND/COM | VIN / DATA IN / COM/GND | VIN / DATA OUT / GND/COM | NLED WS2811 3 Channel / MOSFET Driver v.1a / www.NLEDshop.com/ws2811fet | NLED WS2811 3 Channel / MOSFET Driver v.1a / www.NLEDshop.com/ws2811fet | +5v | +5v | Copyright 2019 / Northern Lights / Electronic Design, LLC | Copyright 2019 / Northern Lights / Electronic Design, LLC | GND | GND | B G R V+ | B G R V+ | 7v-24v | 7v-24v | 7v-24v | 7v-24v | VIN / DATA IN / COM/GND | VIN / DATA OUT / GND/COM | VIN / DATA IN / COM/GND | VIN / DATA OUT / GND/COM | NLED WS2811 3 Channel / MOSFET Driver v.1a / www.NLEDshop.com/ws2811fet | NLED WS2811 3 Channel / MOSFET Driver v.1a / www.NLEDshop.com/ws2811fet | +5v | +5v | Copyright 2019 / Northern Lights / Electronic Design, LLC | Copyright 2019 / Northern Lights / Electronic Design, LLC | GND | GND
_tNames: OUTPUT | OUTPUT | INPUT | INPUT | Q1 | Q2 | Q3 | Q1 | Q2 | Q3 | VREG-B | VREG-B | C1 | C4 | C1 | C4 | RN1 | RN1 | Q4 | Q5 | Q6 | Q4 | Q5 | Q6 | RN3 | WS2811 | RN3 | WS2811 | VREG-A | VREG-A | SPD-J | SPD-J | RN2 | RN2 | C3 | C2 | C3 | C2 | OUTPUT | OUTPUT | INPUT | INPUT | Q1 | Q2 | Q3 | Q1 | Q2 | Q3 | VREG-B | VREG-B | C1 | C4 | C1 | C4 | RN1 | RN1 | Q4 | Q5 | Q6 | Q4 | Q5 | Q6 | RN3 | WS2811 | RN3 | WS2811 | VREG-A | VREG-A | SPD-J | SPD-J | RN2 | RN2 | C3 | C2 | C3 | C2
_bNames: 5VOUT | 5VOUT | 5VOUT | 5VOUT
_tValues: WS2811 | WS2811 | WS2811 | WS2811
